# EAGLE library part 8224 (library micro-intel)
MICROCOMPUTER/PERIPHERAL DEVICE
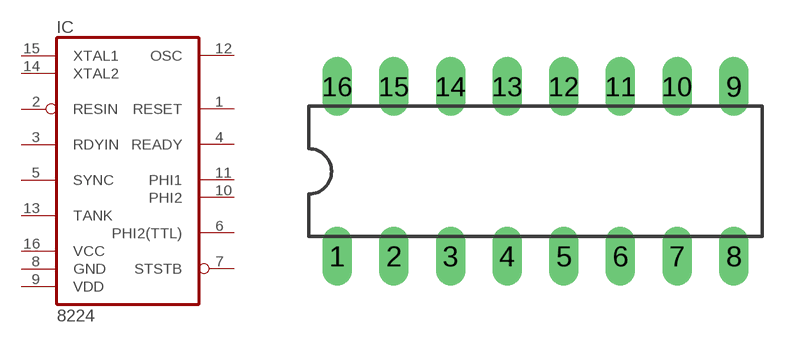
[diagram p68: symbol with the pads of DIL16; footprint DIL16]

Designator prefix IC

## 8224 (OC_FARNELL: unknown; OC_NEWARK: unknown)  [DIL16]
1  RESET  out
2  RESIN  in
3  RDYIN  in
4  READY  out
5  SYNC  in
6  PHI2(TTL)  out
7  STSTB  out
8  GND  pwr
9  VDD  pwr
10  PHI2  out
11  PHI1  out
12  OSC  out
13  TANK  in
14  XTAL2  in
15  XTAL1  in
16  VCC  pwr

## Footprint DIL16 (pad centres in mm)
Dual In Line Package
drill 0.813 long: 1 -8.89,-3.81; 2 -6.35,-3.81; 3 -3.81,-3.81; 4 -1.27,-3.81; 5 1.27,-3.81; 6 3.81,-3.81; 7 6.35,-3.81; 8 8.89,-3.81; 9 8.89,3.81; 10 6.35,3.81; 11 3.81,3.81; 12 1.27,3.81; 13 -1.27,3.81; 14 -3.81,3.81; 15 -6.35,3.81; 16 -8.89,3.81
